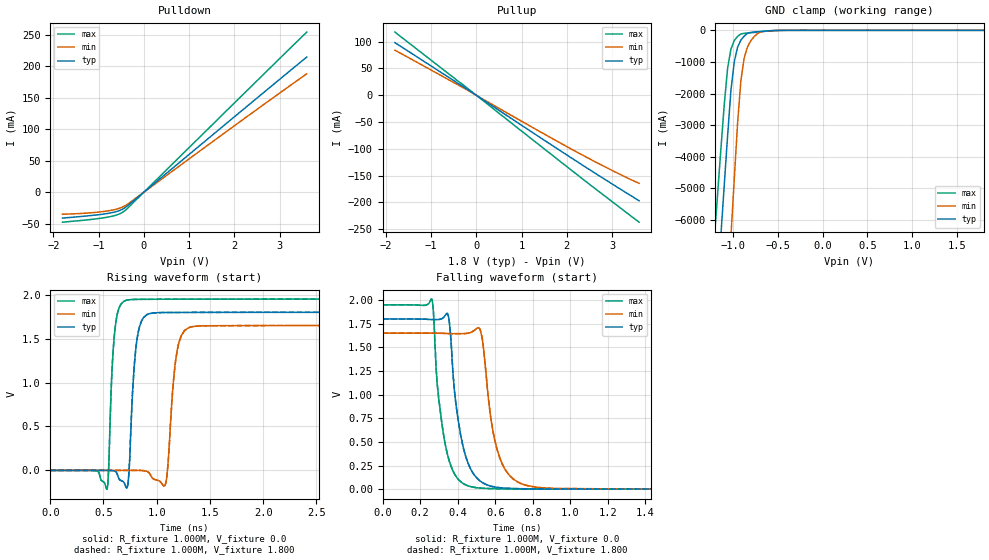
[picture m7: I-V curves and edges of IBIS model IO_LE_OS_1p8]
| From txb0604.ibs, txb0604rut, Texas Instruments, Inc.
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|   Model IO_LE_OS_1p8
[Model] IO_LE_OS_1p8
Model_type 3-state
Polarity   Non-Inverting
Enable   Active-High
Vmeas =  0.900V
Cref =  15.000pF
Rref =  1.000M
Vref =  0.0V
C_comp   3.790pF   3.490pF   3.980pF
[Temperature Range]   27.000   0.125k   -40.000
[Voltage Range]   1.800V   1.650V   1.950V
[Pullup Reference]   1.800V   1.650V   1.950V
[Pulldown Reference]   0.0V   0.0V   0.0V
[POWER Clamp Reference]   1.800V   1.650V   1.950V
[GND Clamp Reference]   0.0V   0.0V   0.0V
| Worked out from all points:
|   slope of the pulldown table from 0 to 0.27 V, typ, clamps not added: 16.7 ohm
|   slope of the pullup table from 0 to 0.27 V, typ, clamps not added: 17.8 ohm
|   GND clamp passes 1 mA (typ) near -0.43 V on its own axis
|   rising waveform, R_fixture 1.000M, V_fixture 0.0: 20-80 % time 55.4ps typ, 66.1ps min, 46ps max; typ from 0 V to 1.8 V
|   rising waveform, R_fixture 1.000M, V_fixture 1.800: 20-80 % time 55.4ps typ, 66.1ps min, 46ps max; typ from 0 V to 1.8 V
|   falling waveform, R_fixture 1.000M, V_fixture 0.0: 20-80 % time 72.5ps typ, 78.3ps min, 64.7ps max; typ from 1.8 V to 0 V
|   falling waveform, R_fixture 1.000M, V_fixture 1.800: 20-80 % time 72.5ps typ, 78.3ps min, 64.7ps max; typ from 1.8 V to 0 V
[Pulldown]
|Voltage   I(typ)   I(min)   I(max)
-1.8V     -41.22mA   -35.02mA   -47.72mA
-1.25V    -37.72mA   -33.2mA    -43.97mA
-810mV    -33.92mA   -29.9mA    -39.77mA
-590mV    -30.52mA   -26.7mA    -35.92mA
-425mV    -25.06mA   -21.86mA   -29.68mA
3.6V      214.7mA    188.1mA    254.4mA
[Pullup]
|Voltage   I(typ)   I(min)   I(max)
-1.8V     98.21mA    84.09mA    117.9mA
-250mV    14.05mA    12.19mA    16.72mA
2.115V    -117.6mA   -101mA     -140.6mA
3.05V     -167.9mA   -142.3mA   -201.5mA
3.6V      -196.8mA   -164.3mA   -236.8mA
[GND_clamp]
|Voltage   I(typ)   I(min)   I(max)
-1.8V     -34.36A    -44.21A    -29.4A
-1.208V   -9.521A    -15.48A    -6.558A
-1.171V   -7.969A    -13.69A    -5.131A
-1.134V   -6.417A    -11.89A    -3.704A
-1.06V    -3.312A    -8.299A    -1.19A
-1.023V   -1.893A    -6.504A    -593mA
-986mV    -994.4mA   -4.708A    -323.1mA
-949mV    -530.7mA   -2.941A    -190.7mA
-912mV    -308.1mA   -1.586A    -114.8mA
-838mV    -95.13mA   -519.5mA   -83.45mA
-653mV    -26.56mA   -29.86mA   -34.54mA
1.8V      0A         0A         0A
[Ramp]
| variable   typ   min   max
dV/dt_r   1.080/55.444p   0.990/66.873p   1.170/45.971p
dV/dt_f   1.080/73.006p   0.990/78.381p   1.170/64.169p
R_load = 1.000M
[Rising Waveform]
R_fixture= 1.000M
V_fixture= 0.0
V_fixture_min= 0.0
V_fixture_max= 0.0
|time   V(typ)   V(min)   V(max)
0s        -25.16nV   2.23uV     -44.26nV
533ps     -30.07uV   -31.4uV    -213.7mV
608ps     -9.756mV   -54.13uV   1.609V
732ps     -133.8mV   -106.2uV   1.941V
809ps     1.441V     -7.923uV   1.946V
960ps     1.791V     -90.18mV   1.948V
1.083ns   1.797V     -152.9mV   1.948V
1.192ns   1.798V     1.362V     1.949V
1.352ns   1.798V     1.64V      1.949V
10ns      1.8V       1.65V      1.95V
[Rising Waveform]
R_fixture= 1.000M
V_fixture= 1.800
V_fixture_min= 1.650
V_fixture_max= 1.950
|time   V(typ)   V(min)   V(max)
0s        29.94uV    33.31uV    27.42uV
533ps     -76.82nV   -320.4nV   -213.7mV
608ps     -9.725mV   -23.05uV   1.609V
732ps     -133.7mV   -75.15uV   1.941V
809ps     1.441V     23.26uV    1.946V
960ps     1.791V     -90.13mV   1.948V
1.083ns   1.797V     -152.8mV   1.948V
1.192ns   1.798V     1.362V     1.949V
1.352ns   1.798V     1.64V      1.949V
10ns      1.8V       1.65V      1.95V
[Falling Waveform]
R_fixture= 1.000M
V_fixture= 0.0
V_fixture_min= 0.0
V_fixture_max= 0.0
|time   V(typ)   V(min)   V(max)
0s        1.8V       1.65V      1.95V
264ps     1.794V     1.65V      2V
289ps     1.794V     1.65V      1.144V
345ps     1.858V     1.646V     368.3mV
414ps     587.5mV    1.645V     82.06mV
512ps     98.64mV    1.706V     12.73mV
587ps     27.23mV    619.4mV    5.267mV
626ps     15mV       320.9mV    4.045mV
826ps     3.084mV    18.09mV    2.142mV
10ns      8.725uV    19.14uV    3.619uV
[Falling Waveform]
R_fixture= 1.000M
V_fixture= 1.800
V_fixture_min= 1.650
V_fixture_max= 1.950
|time   V(typ)   V(min)   V(max)
0s        1.8V       1.65V      1.95V
264ps     1.794V     1.65V      2V
289ps     1.794V     1.65V      1.144V
345ps     1.858V     1.647V     368.3mV
414ps     587.5mV    1.645V     82.09mV
512ps     98.67mV    1.706V     12.76mV
587ps     27.25mV    619.5mV    5.294mV
626ps     15.03mV    320.9mV    4.073mV
826ps     3.114mV    18.12mV    2.17mV
10ns      38.69uV    50.22uV    31.08uV
